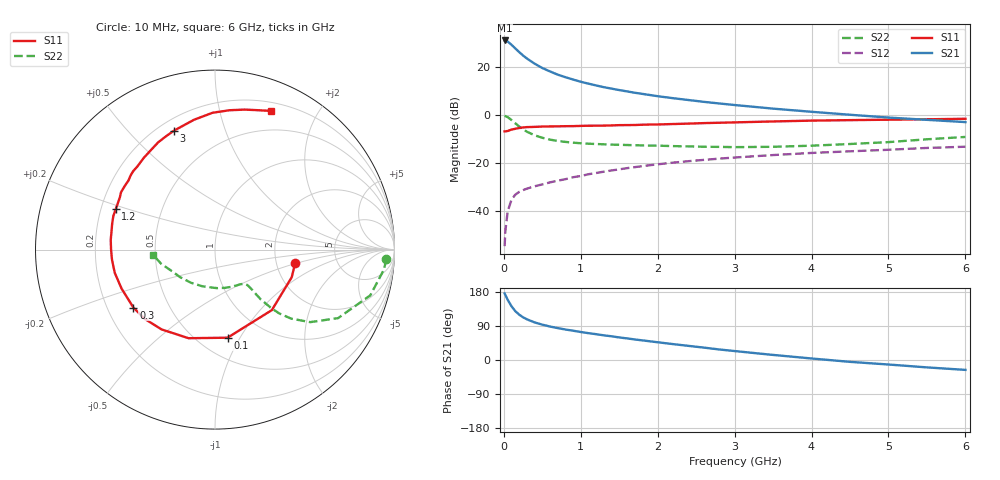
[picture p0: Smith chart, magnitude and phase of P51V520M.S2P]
! SIEMENS Small Signal Semiconductors
! BFP183
! Si NPN RF Bipolar Junction Transistor in SOT143
! VCE = 1.5 V  IC = 20 mA
! Common Emitter S-Parameters:  March  1996
# GHz  S  MA  R  50
!  f  S11  S21  S12  S22
! GHz  MAG  ANG  MAG  ANG  MAG  ANG  MAG  ANG
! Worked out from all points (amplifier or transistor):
!   36 points, 10 MHz to 6 GHz, reference 50 ohm
!   highest |S21| = 31.2 dB at 10 MHz (marker M1)
!   |S21| within 3 dB of that: start of sweep to 138.2 MHz
!   unconditionally stable (mu >= 1): 679.9 MHz to 5.853 GHz
!   at 250 MHz: K = 0.53, MSG = 28.2 dB, |S12| = -31.4 dB
!   at 1.4 GHz: K = 1.20, MAG = 14.4 dB, |S12| = -23.2 dB
!   at 6 GHz: K = 0.98, MSG = 5.1 dB, |S12| = -13.3 dB
!   S11 on the Smith chart (normalised r, x): 10 MHz: 2.55, -0.48; 100 MHz: 0.68, -0.89; 300 MHz: 0.31, -0.29; 1.2 GHz: 0.26, +0.18; 3 GHz: 0.26, +0.68; 6 GHz: 0.29, +1.44
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0.01  0.4531 -9.6  36.29 175.7  0.0018 84.8  0.9557 -3.2
0.02  0.4544 -19.8  36.14 171.6  0.0038 78.1  0.948 -6.7
0.05  0.4626 -46.8  34.45 158.8  0.0096 75.2  0.9021 -16.4
0.1  0.4958 -81.9  29.43 141.7  0.017 61.4  0.7849 -29.1
0.15  0.5152 -106.6  24.64 128.7  0.0216 54.3  0.6669 -37.3
0.2  0.5351 -123.8  20.68 119.6  0.0246 50.0  0.5725 -42.2
0.25  0.5498 -135.4  17.56 112.7  0.0268 47.7  0.5021 -44.9
0.3  0.5577 -144.6  15.21 107.4  0.0288 46.9  0.4472 -46.2
0.4  0.564 -157.3  11.85 99.2  0.0322 47.2  0.3764 -47.4
0.5  0.5733 -166.9  9.622 93.3  0.0353 47.6  0.3335 -47.4
0.6  0.5767 -174.4  8.159 88.3  0.0389 49.3  0.3054 -47.3
0.7  0.5791 179.8  6.991 84.2  0.0422 50.5  0.2862 -47.3
0.8  0.5834 174.7  6.181 80.5  0.0454 51.4  0.2734 -47.4
1.1  0.5966 161.7  4.529 70.8  0.0576 53.1  0.251 -49.6
1.2  0.5971 157.8  4.148 68.1  0.0611 53.0  0.2471 -50.6
1.7  0.6169 141.4  2.925 54.3  0.081 51.7  0.2334 -58.8
2.2  0.6472 127.8  2.248 41.9  0.1007 48.4  0.2233 -69.9
3  0.7008 109.1  1.618 23.6  0.1289 41.7  0.2125 -92.7
3.5  0.7327 99.2  1.359 13.4  0.1451 37.2  0.2162 -109.0
4.5  0.7808 84.0  1.012 -4.9  0.1738 28.1  0.2473 -141.5
5.5  0.8126 72.9  0.792 -19.5  0.2045 20.0  0.3103 -165.3
6  0.8333 68.0  0.71 -26.1  0.2169 15.3  0.3474 -175.4
